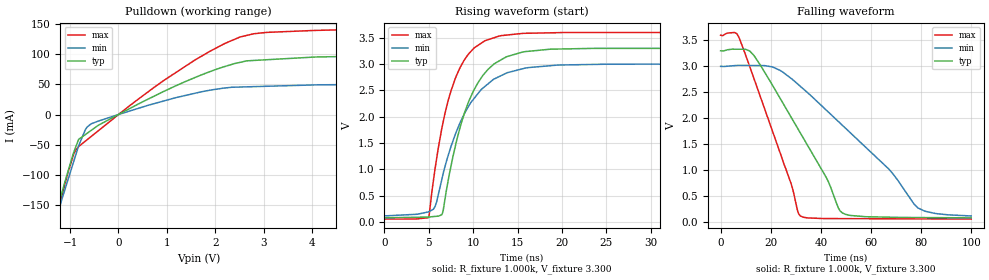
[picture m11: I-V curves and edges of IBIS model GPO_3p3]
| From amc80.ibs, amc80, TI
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|   GPO model
[Model]  GPO_3p3
Model_type   Open_drain
Polarity   Non-Inverting
Vmeas = 1.65
Vref = 1.65
Cref = 15pF
Rref = 50
|   typ   min   max
|   (nom PVT)   (Fast PVT)   (slow PVT)
|   ON state : BUFFER OUTPUT TURNED HIGH
|C_comp   1.265E-12   1.028E-12   1.459E-12
|   OFF state: BUFFER OUTPUT TURNED LOW
C_comp   9.685E-13   9.249E-13   1.072E-12
| Where   nom PVT is  Nominal Process, 3.3V, 27C
|   Fast PVT is Strong Process, 3.6V, -40C
|   Slow PVT is Weak Process, 3.0V, 125C
|C_comp - from L-C Tank method, L = 1nH, peak frequency
[Voltage Range]   3.3   3   3.6
[Temperature Range]   27   125   -40
[Pullup Reference]   3.3   3   3.6
[Pulldown Reference]   0   0   0
[Power Clamp Reference]   3.3   3   3.6
[GND Clamp Reference]   0   0   0
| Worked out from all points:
|   slope of the pulldown table from 0 to 0.495 V, typ, clamps not added: 23.7 ohm
|   falling waveform, R_fixture 1.000k, V_fixture 3.300: 20-80 % time 23ns typ, 36ns min, 15.6ns max; typ from 3.3 V to 0.08 V
|   rising waveform, R_fixture 1.000k, V_fixture 3.300: 20-80 % time 3.46ns typ, 4.15ns min, 2.9ns max; typ from 0.08 V to 3.3 V
[Pulldown]
|   Voltage   I(typ)   I(min)   I(max)
-3.3V     -814.3mA   -776mA     -897.8mA
-1.355V   -184.2mA   -192.7mA   -192.2mA
-1.164V   -128.3mA   -139mA     -133.2mA
-916.3mV  -60.81mA   -75.51mA   -63.95mA
-824.8mV  -41.33mA   -52.07mA   -53.51mA
-683.5mV  -33.19mA   -24.88mA   -44.14mA
-564.1mV  -26.33mA   -15.38mA   -36.44mA
929.8mV   38.06mA    22.3mA     56.04mA
1.893V    71.16mA    40.31mA    105mA
2.518V    86.56mA    45.59mA    128.7mA
3.062V    90.84mA    46.82mA    136.2mA
6.59V     98.58mA    50.8mA     144.3mA
[Ramp]
R_load = 1000
|   typ   min   max
dV/dt_r   1.93221/3.46605e-009   1.70385/4.10522e-009   2.12618/2.9023e-009
dV/dt_f   1.93221/2.30081e-008   1.70385/3.59901e-008   2.12618/1.5543e-008
[Falling Waveform]
R_fixture = 1.000k
V_fixture = 3.300
V_fixture_min = 3.000
V_fixture_max = 3.600
C_fixture = 0.000
|  time   V(typ)   V(min)   V(max)
0s        3.3V       3V         3.6V
7.302ns   3.33V      3.019V     3.559V
13.48ns   3.197V     3.016V     2.741V
23.66ns   2.391V     2.924V     1.345V
31.81ns   1.716V     2.615V     117.8mV
42.29ns   846.1mV    2.15V      65.72mV
48.71ns   171.5mV    1.858V     64.68mV
67.14ns   92.41mV    1.019V     61.69mV
78.87ns   85.45mV    267.5mV    59.79mV
100ns     79.66mV    115.7mV    56.37mV
[Rising Waveform]
R_fixture = 1.000k
V_fixture = 3.300
V_fixture_min = 3.000
V_fixture_max = 3.600
C_fixture = 0.000
|  time   V(typ)   V(min)   V(max)
0s        79.66mV    115.7mV    56.37mV
4.976ns   95.38mV    192.6mV    81.55mV
5.721ns   106.5mV    297mV      1.017V
6.494ns   141.8mV    819.9mV    1.792V
8.016ns   1.452V     1.675V     2.735V
9.51ns    2.293V     2.204V     3.196V
11.05ns   2.774V     2.536V     3.411V
12.97ns   3.063V     2.765V     3.533V
23.65ns   3.298V     2.993V     3.599V
100ns     3.3V       3V         3.6V
